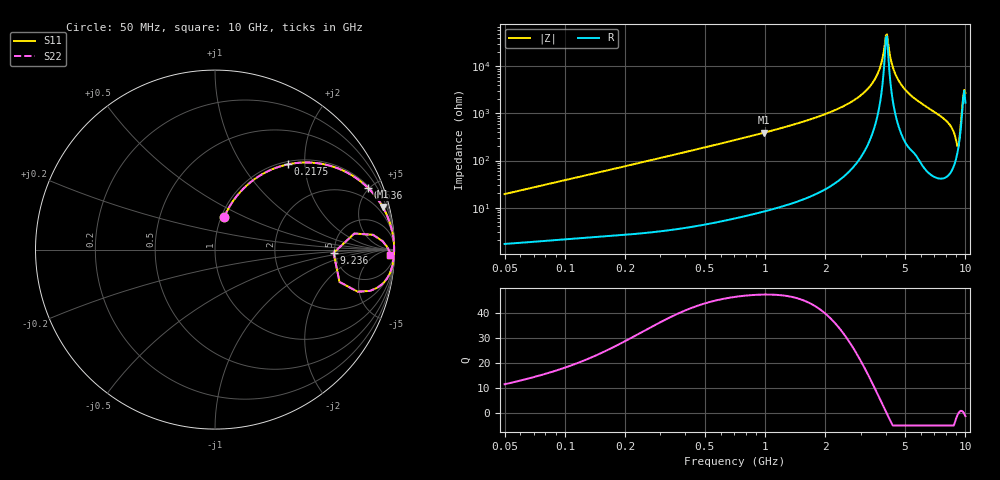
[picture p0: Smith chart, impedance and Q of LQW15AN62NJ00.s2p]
!Murata Part Number: LQW15AN62NJ00
!These Parameters are Measured in Series Mode Connection
!  o--[Z]--o
!Port1  Port2
!  o-------o
!Freq. Start=50[MHz] Stop=10[GHz], 401[Steps]
# Hz S RI R 50
!Freq.(Hz)	S 11(Real)	S 11(Imag)	S 21(Real)	S 21(Imag)	S 12(Real)	S 12(Imag)	S 22(Real)	S 22(Imag)
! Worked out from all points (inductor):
!   401 points, 50 MHz to 10 GHz, reference 50 ohm
!   read as one part in series: L = 61.2 nH near 51.34 MHz
!   highest Q = 47.3 at 984.7 MHz (marker M1), where L = 62.9 nH
!   self-resonance near 4.009 GHz
!   S11 on the Smith chart (normalised r, x): 50 MHz: 1.03, +0.39; 217.5 MHz: 1.05, +1.65; 636 MHz: 1.11, +4.88; 9.236 GHz: 4.88, -0.32; 10 GHz: 35, -43
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5e7  0.0509 0.1803  0.9491 -0.1803  0.9491 -0.1803  0.0509 0.1803
1.214486e8  0.1878 0.367  0.8122 -0.367  0.8122 -0.367  0.1878 0.367
2.175233e8  0.4073 0.4751  0.5927 -0.4751  0.5927 -0.4751  0.4073 0.4751
2.949953e8  0.5535 0.4834  0.4465 -0.4834  0.4465 -0.4834  0.5535 0.4834
6.360107e8  0.8508 0.3456  0.1492 -0.3456  0.1492 -0.3456  0.8508 0.3456
7.071068e8  0.8761 0.3189  0.1239 -0.3189  0.1239 -0.3189  0.8761 0.3189
9.846897e8  0.9338 0.2384  0.0662 -0.2384  0.0662 -0.2384  0.9338 0.2384
1.717543e9  0.9807 0.1264  0.0193 -0.1264  0.0193 -0.1264  0.9807 0.1264
2.423676e9  0.9926 0.0715  0.00737 -0.0715  0.00737 -0.0715  0.9926 0.0715
3.076244e9  0.9966 0.0375  0.00337 -0.0375  0.00337 -0.0375  0.9966 0.0375
3.654301e9  0.9979 0.0138  0.00208 -0.0138  0.00208 -0.0138  0.9979 0.0138
4.009335e9  0.9981 0.00103  0.00191 -0.00103  0.00191 -0.00103  0.9981 0.00103
4.116968e9  0.9981 -0.00266  0.00194 0.00266  0.00194 0.00266  0.9981 -0.00266
4.171863e9  0.998 -0.00451  0.00196 0.00451  0.00196 0.00451  0.998 -0.00451
4.457516e9  0.9978 -0.0139  0.00221 0.0139  0.00221 0.0139  0.9978 -0.0139
4.955797e9  0.9968 -0.0294  0.00318 0.0294  0.00318 0.0294  0.9968 -0.0294
7.878683e9  0.9753 -0.1292  0.0247 0.1292  0.0247 0.1292  0.9753 -0.1292
8.759398e9  0.9033 -0.2129  0.0967 0.2129  0.0967 0.2129  0.9033 -0.2129
8.994549e9  0.7949 -0.2347  0.2051 0.2347  0.2051 0.2347  0.7949 -0.2347
9.236013e9  0.6608 -0.0183  0.3392 0.0183  0.3392 0.0183  0.6608 -0.0183
9.738562e9  0.9583 0.0161  0.0417 -0.0161  0.0417 -0.0161  0.9583 0.0161
1e10  0.977 -0.0275  0.023 0.0275  0.023 0.0275  0.977 -0.0275
